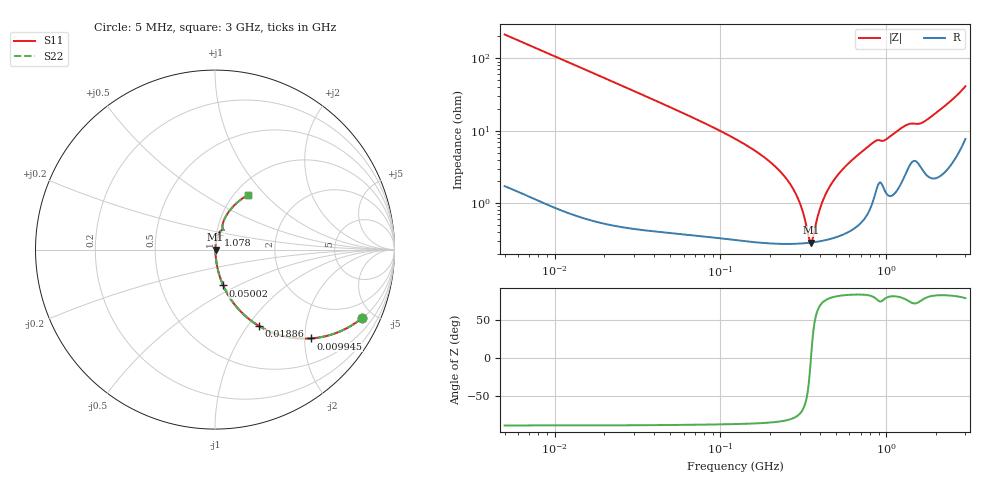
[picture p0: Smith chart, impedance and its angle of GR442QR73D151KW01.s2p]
!Murata Part Number: GR442QR73D151KW01
!These Parameters are Measured in Series Mode Connection
!Data Generated on Mar 13, 2026
!  o--ll--o
!Port1  Port2
!  o------o
!Operation Temp=25[degC], DC Bias Voltage=0[V]
!Freq. Start=5[MHz] Stop=3[GHz] 401[Steps]
# Hz S RI R 50
!Freq.(Hz) S11(Real) S11(Imag) S21(Real) S21(Imag) S12(Real) S12(Imag) S22(Real) S22(Imag)
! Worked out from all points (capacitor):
!   401 points, 5 MHz to 3 GHz, reference 50 ohm
!   read as one part in series: C = 150 pF near 5.163 MHz
!   lowest |Z| = 286 mohm at 351.9 MHz (marker M1)
!   series resonance near 351.6 MHz, so ESL is about 1.4 nH
!   S11 on the Smith chart (normalised r, x): 5 MHz: 1.03, -4.25; 9.945 MHz: 1.02, -2.14; 18.86 MHz: 1.01, -1.13; 50.02 MHz: 1.01, -0.42; 1.078 GHz: 1.03, +0.17; 3 GHz: 1.15, +0.81
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5000000  0.8166 -0.3829  0.1834 0.3829  0.1834 0.3829  0.8166 -0.3829
9945377  0.534 -0.4948  0.466 0.4948  0.466 0.4948  0.534 -0.4948
1.459857e7  0.3487 -0.4723  0.6513 0.4723  0.6513 0.4723  0.3487 -0.4723
1.885543e7  0.2438 -0.4247  0.7562 0.4247  0.7562 0.4247  0.2438 -0.4247
4.262365e7  0.061 -0.2313  0.939 0.2313  0.939 0.2313  0.061 -0.2313
5.001548e7  0.0455 -0.1995  0.9545 0.1995  0.9545 0.1995  0.0455 -0.1995
1.244489e8  0.00874 -0.075  0.9913 0.075  0.9913 0.075  0.00874 -0.075
1.886127e8  0.00446 -0.0407  0.9955 0.0407  0.9955 0.0407  0.00446 -0.0407
2.515288e8  0.00318 -0.021  0.9968 0.021  0.9968 0.021  0.00318 -0.021
2.951491e8  0.00288 -0.0109  0.9971 0.0109  0.9971 0.0109  0.00288 -0.0109
3.408394e8  0.00283 -0.00193  0.9972 0.00193  0.9972 0.00193  0.00283 -0.00193
3.519173e8  0.00285 5.2e-05  0.9971 -5.2e-05  0.9971 -5.2e-05  0.00285 5.2e-05
3.575905e8  0.00287 0.00105  0.9971 -0.00105  0.9971 -0.00105  0.00287 0.00105
4.12947e8  0.00312 0.0101  0.9969 -0.0101  0.9969 -0.0101  0.00312 0.0101
5.003097e8  0.00391 0.0227  0.9961 -0.0227  0.9961 -0.0227  0.00391 0.0227
8.213828e8  0.0139 0.0645  0.9861 -0.0645  0.9861 -0.0645  0.0139 0.0645
1.044062e9  0.0187 0.0785  0.9813 -0.0785  0.9813 -0.0785  0.0187 0.0785
1.077996e9  0.0196 0.0832  0.9804 -0.0832  0.9804 -0.0832  0.0196 0.0832
1.32711e9  0.039 0.1094  0.961 -0.1094  0.961 -0.1094  0.039 0.1094
1.686893e9  0.0416 0.1214  0.9584 -0.1214  0.9584 -0.1214  0.0416 0.1214
2.322711e9  0.0744 0.2074  0.9256 -0.2074  0.9256 -0.2074  0.0744 0.2074
3e9  0.1852 0.3046  0.8148 -0.3046  0.8148 -0.3046  0.1852 0.3046
